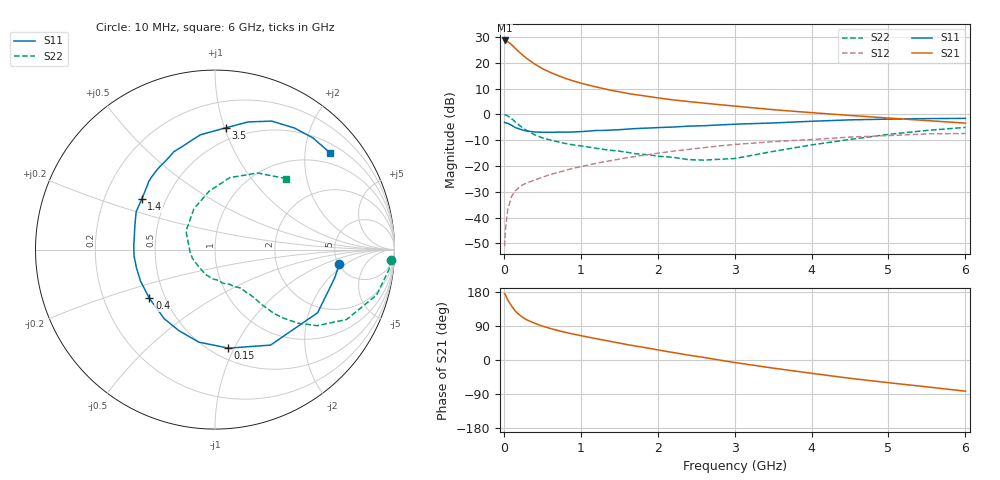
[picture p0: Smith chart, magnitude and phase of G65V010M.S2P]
! SIEMENS Small Signal Semiconductors
! BFG193
! Si NPN RF Bipolar Junction Transistor in SOT223
! VCE = 5 V  IC = 10 mA
! Common Emitter S-Parameters:  August  1996
# GHz  S  MA  R  50
!  f  S11  S21  S12  S22
! GHz  MAG  ANG  MAG  ANG  MAG  ANG  MAG  ANG
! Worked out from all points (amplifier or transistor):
!   36 points, 10 MHz to 6 GHz, reference 50 ohm
!   highest |S21| = 28.6 dB at 10 MHz (marker M1)
!   |S21| within 3 dB of that: start of sweep to 146.6 MHz
!   unconditionally stable (mu >= 1): 884.8 MHz to 2.488 GHz
!   at 250 MHz: K = 0.53, MSG = 25.0 dB, |S12| = -27.2 dB
!   at 1.4 GHz: K = 1.07, MAG = 12.0 dB, |S12| = -17.9 dB
!   at 6 GHz: K = 0.87, MSG = 2.0 dB, |S12| = -7.4 dB
!   S11 on the Smith chart (normalised r, x): 10 MHz: 5.11, -1.57; 150 MHz: 0.60, -0.95; 400 MHz: 0.41, -0.28; 1.4 GHz: 0.37, +0.27; 3.5 GHz: 0.40, +1.01; 6 GHz: 0.71, +2.57
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0.01  0.6975 -6.5  27.01 175.3  0.0028 93.9  0.9822 -3.3
0.02  0.6854 -13.3  26.89 171.8  0.0055 80.9  0.976 -6.5
0.05  0.6714 -31.6  25.63 158.6  0.0143 76.7  0.9353 -15.7
0.1  0.6156 -59.8  22.46 142.8  0.0256 65.8  0.8299 -28.0
0.15  0.5539 -82.4  18.9 128.7  0.0332 57.6  0.7092 -36.7
0.2  0.5232 -100.0  16.15 119.6  0.0389 54.7  0.6184 -41.5
0.25  0.4939 -114.2  13.83 111.8  0.0435 51.8  0.5387 -45.1
0.3  0.4779 -126.3  12.03 105.8  0.0471 51.4  0.4845 -47.3
0.4  0.4554 -143.4  9.469 97.1  0.0535 50.5  0.4022 -49.6
0.5  0.4505 -157.2  7.714 89.4  0.0604 50.1  0.3524 -50.7
0.6  0.4492 -166.9  6.556 83.4  0.0682 51.3  0.3202 -52.0
0.7  0.4525 -175.7  5.684 78.0  0.0747 51.4  0.2951 -53.8
0.9  0.4555 170.7  4.459 68.5  0.0903 50.9  0.257 -56.4
1.1  0.4742 159.2  3.683 60.3  0.1044 49.9  0.2332 -62.3
1.4  0.4957 145.6  2.907 48.5  0.1277 46.9  0.2009 -71.4
1.7  0.5291 134.3  2.425 37.3  0.1523 43.1  0.1737 -82.7
2.2  0.5683 118.2  1.907 19.8  0.1938 34.3  0.1472 -112.0
2.8  0.6236 101.8  1.544 0.0  0.2446 22.7  0.1349 -158.9
3.5  0.6814 84.9  1.233 -21.4  0.2956 6.9  0.1917 147.4
4.5  0.7825 66.2  0.953 -48.3  0.3633 -12.9  0.3267 95.8
5.5  0.8276 48.7  0.758 -70.9  0.4183 -37.4  0.4887 60.8
6  0.8372 40.1  0.677 -82.3  0.4261 -51.4  0.5595 45.0
